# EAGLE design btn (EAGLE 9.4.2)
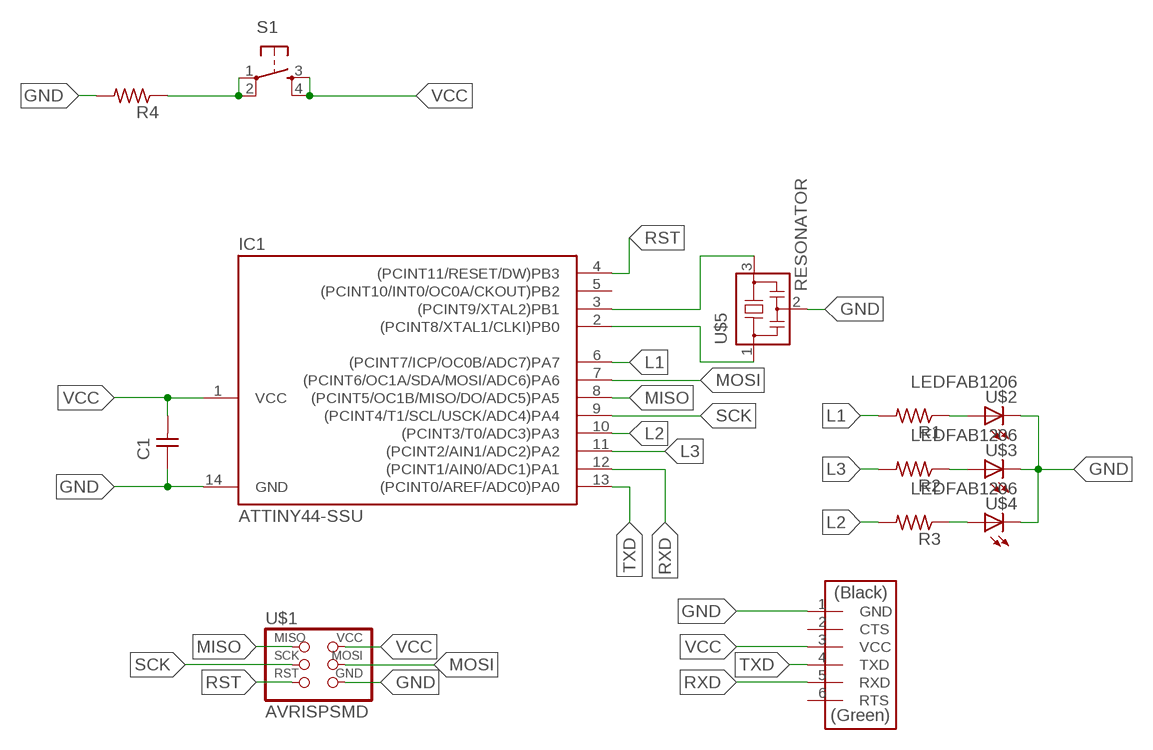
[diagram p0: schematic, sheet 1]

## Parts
C1  CAP-UNPOLARIZEDFAB  [C1206FAB]
IC1  ATTINY44-SSU  [SOIC14]
R1  RES-US1206FAB  [R1206FAB]
R2  RES-US1206FAB  [R1206FAB]
R3  RES-US1206FAB  [R1206FAB]
R4  RES-US1206FAB  [R1206FAB]
S1  6MM_SWITCH6MM_SWITCH  [6MM_SWITCH]
U$1  AVRISPSMD  [2X03SMD]
U$2  LEDFAB1206  [LED1206FAB]
U$3  LEDFAB1206  [LED1206FAB]
U$4  LEDFAB1206  [LED1206FAB]
U$5  RESONATOR  [EFOBM]
U$6  FTDI-SMD-HEADER  [1X06SMD]

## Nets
GND: C1.1 IC1.14(GND) R4.2 U$1.6(GND) U$2.2(C) U$3.2(C) U$4.2(C) U$5.2 U$6.1(GND)
L1: IC1.6((PCINT7/ICP/OC0B/ADC7)PA7) R1.2
L2: IC1.10((PCINT3/T0/ADC3)PA3) R3.2
L3: IC1.11((PCINT2/AIN1/ADC2)PA2) R2.2
MISO: IC1.8((PCINT5/OC1B/MISO/DO/ADC5)PA5) U$1.1(MISO)
MOSI: IC1.7((PCINT6/OC1A/SDA/MOSI/ADC6)PA6) U$1.4(MOSI)
N$1: IC1.3((PCINT9/XTAL2)PB1) U$5.3
N$2: IC1.2((PCINT8/XTAL1/CLKI)PB0) U$5.1
N$4: R1.1 U$2.1(A)
N$5: R2.1 U$3.1(A)
N$6: R3.1 U$4.1(A)
N$21: R4.1 S1.1(P) S1.2(P1)
RST: IC1.4((PCINT11/RESET/DW)PB3) U$1.5(RST)
RXD: IC1.12((PCINT1/AIN0/ADC1)PA1) U$6.5(RXD)
SCK: IC1.9((PCINT4/T1/SCL/USCK/ADC4)PA4) U$1.3(SCK)
TXD: IC1.13((PCINT0/AREF/ADC0)PA0) U$6.4(TXD)
VCC: C1.2 IC1.1(VCC) S1.3(S) S1.4(S1) U$1.2(VCC) U$6.3(VCC)
Unconnected: IC1.5((PCINT10/INT0/OC0A/CKOUT)PB2) U$6.2(CTS) U$6.6(RTS)

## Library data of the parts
C1 = fab:CAP-UNPOLARIZED
IC1 = fab:ATTINY44
R1-R4 = fab:RES-US: Resistor (US Symbol)
S1 = fab:6MM_SWITCH: OMRON SWITCH
U$1 = fab:AVRISP
U$2-U$4 = fab:LED: LED
U$5 = fab:RESONATOR
U$6 = fab:FTDI-SMD-HEADER

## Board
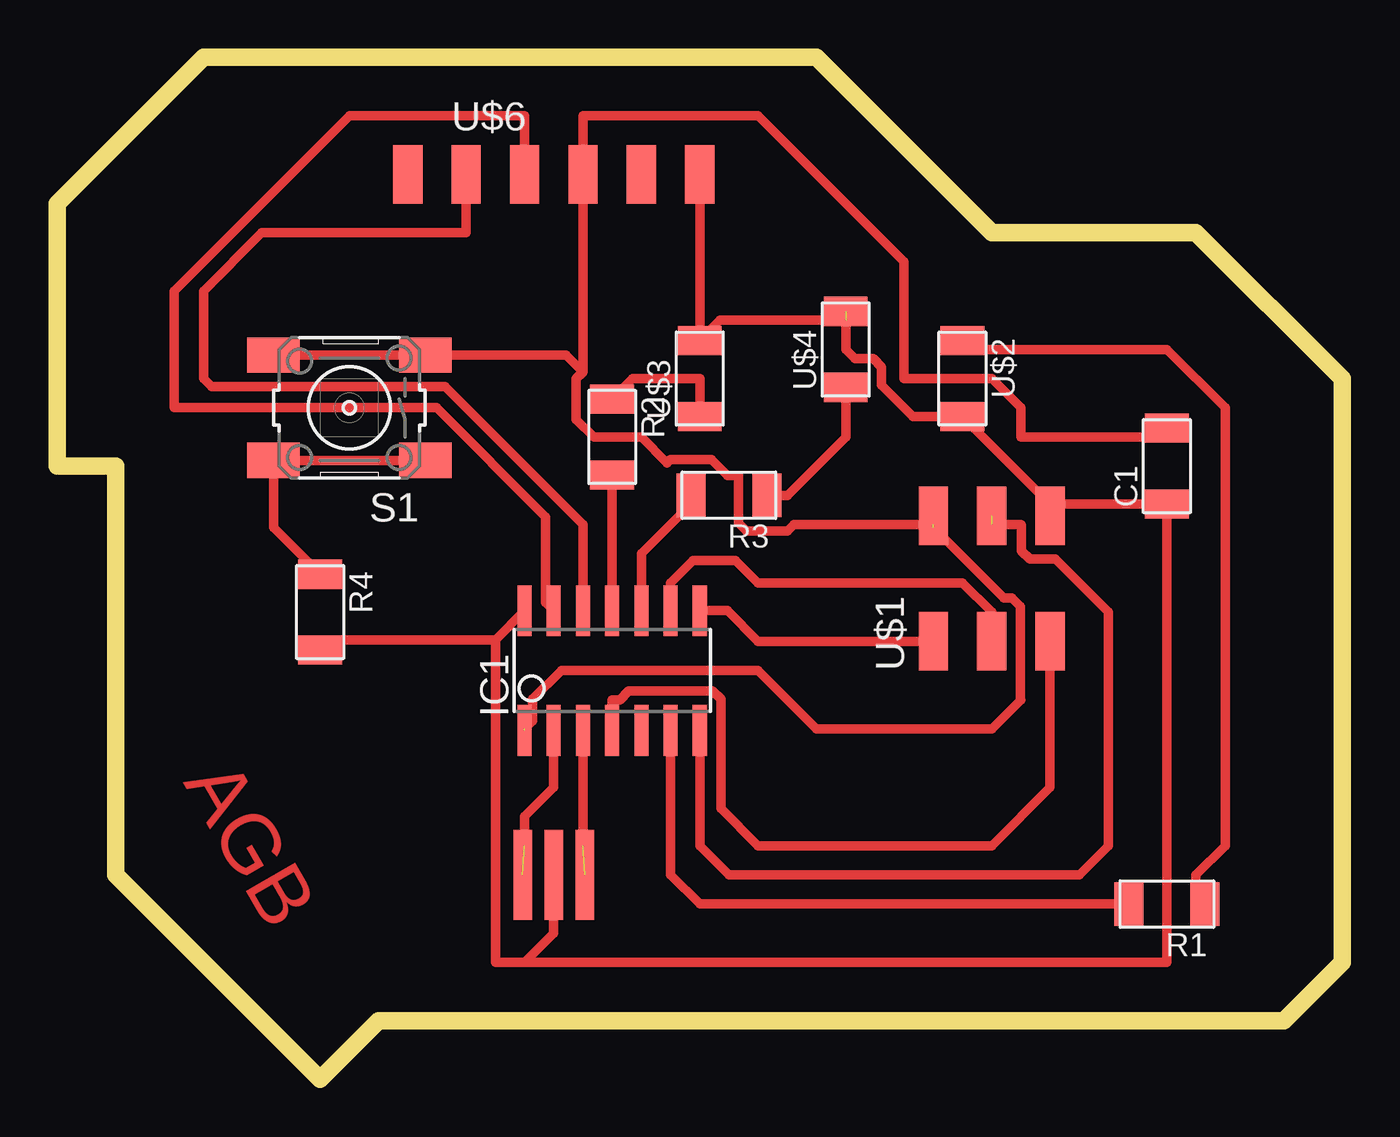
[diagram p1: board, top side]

Size 55.88 x 44.45 mm. Coordinates in mm from the lower left corner, seen from the top.
Outline: 6.35,44.45 33.02,44.45 40.64,36.83 49.53,36.83 55.88,30.48 55.88,5.08 53.34,2.54 13.97,2.54 11.43,0 2.54,8.89 2.54,26.67 0,26.67 0,38.1 6.35,44.45
Copper layers (1*16): Top 0.035mm / dielectric 1.5mm / Bottom 0.035mm
Design rules "default *": minimum track width 16mil, minimum drill 0.35mm, track to track 16mil, track to pad 16mil, pad to pad 16mil, via to via 16mil, smd to smd 16mil, copper to edge 16mil, drill to drill 16mil, minimum pad ring 10mil, minimum via ring 8mil, stop-mask expansion 4mil, vias tented up to drill 0mil, thermal gap 10mil

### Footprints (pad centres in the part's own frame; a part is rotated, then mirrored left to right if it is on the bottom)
C1206FAB = smd 1.27 x 1.905: 1 -1.651,0; 2 1.651,0
SOIC14 = smd 0.61 x 2.21: 1 -3.81,-2.603; 2 -2.54,-2.603; 3 -1.27,-2.603; 4 0,-2.603; 5 1.27,-2.603; 6 2.54,-2.603; 7 3.81,-2.603; 8 3.81,2.603; 9 2.54,2.603; 10 1.27,2.603; 11 0,2.603; 12 -1.27,2.603; 13 -2.54,2.603; 14 -3.81,2.603
R1206FAB = smd 1.27 x 1.905: 1 -1.651,0; 2 1.651,0
6MM_SWITCH = smd 2.286 x 1.524: 1 -3.302,2.286; 2 3.302,2.286; 3 -3.302,-2.286; 4 3.302,-2.286
2X03SMD = smd 2.54 x 1.27: 1 -2.54,2.54; 2 2.92,2.54; 3 -2.54,0; 4 2.92,0; 5 -2.54,-2.54; 6 2.92,-2.54
LED1206FAB = smd 1.27 x 1.905: 1 -1.651,0; 2 1.651,0
EFOBM = smd 0.8 x 3.9: 1 -1.35,0; 2 0,0; 3 1.35,0
1X06SMD = smd 2.54 x 1.27: 1 0,6.35; 2 0,3.81; 3 0,1.27; 4 0,-1.27; 5 0,-3.81; 6 0,-6.35

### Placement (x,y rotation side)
C1  48.26,26.67 90 top
IC1  24.13,17.78 0 top
R1  48.26,7.62 180 top
R2  24.13,27.94 270 top
R3  29.21,25.4 180 top
R4  11.43,20.32 270 top
S1  12.7,29.21 180 top
U$1  40.64,21.59 90 top
U$2  39.37,30.48 270 top
U$3  27.94,30.48 90 top
U$4  34.29,31.75 90 top
U$5  21.59,8.89 0 top
U$6  21.59,39.37 270 top

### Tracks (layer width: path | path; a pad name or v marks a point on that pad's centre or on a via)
GND  (1 unrouted)
  Top 0.406: IC1.14 19.05,19.11 | 20.32,5.08 19.05,5.08 19.05,19.11 | U$5.2 21.59,6.35 20.32,5.08 | 19.05,19.11 11.87,19.11 R4.2 | U$6.1 U$3.2 28.83,33.02 34.29,33.02 | 38.48,28.83 U$2.2 | U$2.2 43.18,25.02 U$1.6 43.69,25.02 C1.1 48.26,5.08 20.32,5.08 | U$2.2 37.21,28.83 35.85,30.19 35.85,30.99 35.49,31.34 34.7,31.34 34.29,31.75 U$4.2
L1
  Top 0.406: R1.2 27.94,7.62 26.67,8.89 IC1.6
L2
  Top 0.406: IC1.10 25.4,22.86 27.56,25.02 R3.2
L3
  Top 0.406: IC1.11 R2.2
MISO
  Top 0.406: IC1.8 29.15,20.38 30.48,19.05 U$1.1
MOSI  (1 unrouted)
  Top 0.406: IC1.7 27.94,10.16 29.21,8.89 44.45,8.89 45.72,10.16 45.72,20.32 43.41,22.63 42.29,22.63 41.94,22.99 41.94,24.11 41.91,24.13 40.64,24.13
N$1  (1 unrouted)
  Top 0.406: IC1.3 22.86,10.16
N$2  (1 unrouted)
  Top 0.406: IC1.2 21.59,12.7 20.32,11.43 20.32,10.16
N$4
  Top 0.406: U$2.1 39.75,31.75 48.26,31.75 50.8,29.21 50.8,10.16 49.53,8.89 49.53,8 R1.1
N$5
  Top 0.406: U$3.1 27.94,30.48 25.02,30.48 R2.1
N$6
  Top 0.406: U$4.1 34.29,27.94 31.75,25.4 R3.1
N$21
  Top 0.406: S1.1 S1.2 9.4,24 R4.1
RST
  Top 0.406: IC1.4 24.13,16.51 24.46,16.51 24.84,16.89 28.5,16.89 28.85,16.53 28.85,11.79 30.48,10.16 40.64,10.16 43.18,12.7 U$1.5
RXD
  Top 0.406: IC1.12 22.86,24.13 16.87,30.12 6.71,30.12 6.35,30.48 6.35,34.29 8.89,36.83 17.78,36.83 U$6.5
SCK
  Top 0.406: IC1.9 26.67,21.59 27.65,22.57 29.5,22.57 30.48,21.59 39.37,21.59 40.64,20.32 U$1.3
TXD
  Top 0.406: IC1.13 21.23,20.74 21.23,24.46 16.48,29.21 5.08,29.21 5.08,34.29 12.7,41.91 20.32,41.91 U$6.4
VCC  (2 unrouted)
  Top 0.406: S1.4 S1.3 | S1.3 16.26,31.75 | 22.86,30.77 U$6.3 22.86,41.91 30.48,41.91 36.83,35.56 36.83,30.48 40.64,30.48 41.91,29.21 41.91,27.94 47.88,27.94 C1.2 | 22.86,30.77 22.57,30.48 22.57,28.7 23.33,27.94 25.4,27.94 26.53,26.82 26.67,26.96 28.45,26.96 29.14,26.26 29.62,26.26 29.62,24.19 29.97,23.84 31.75,23.84 32.04,24.13 38.1,24.13 | U$1.2 38.1,24.01 41.18,20.93 41.53,20.93 41.88,20.57 41.88,16.54 41.91,16.51 40.64,15.24 33.02,15.24 30.48,17.78 21.92,17.78 20.68,16.53 20.68,15.6 20.32,15.24 | S1.3 22.14,31.5 22.86,30.77

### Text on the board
Top: AGB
